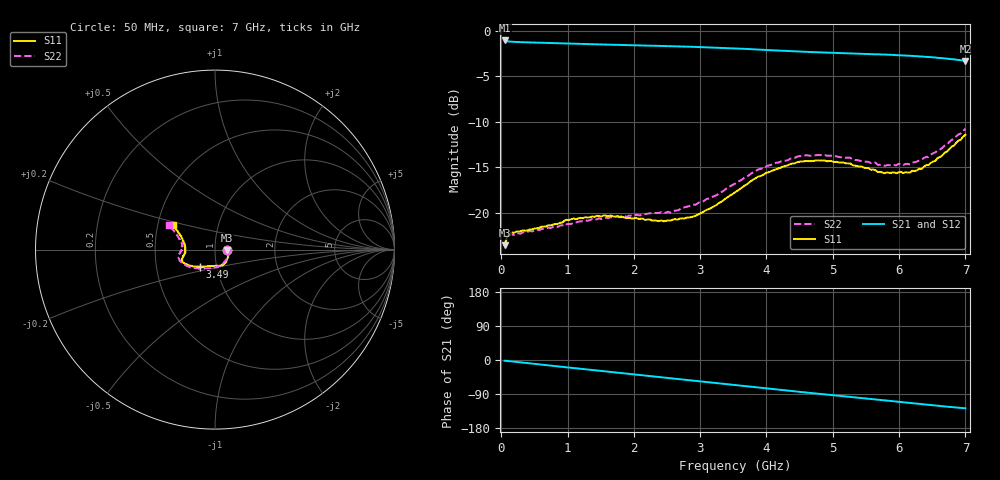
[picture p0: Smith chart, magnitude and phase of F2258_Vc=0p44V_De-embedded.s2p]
! Integrated Device Technology
! Corporate Headquarters
! 6024 Silver Creek Valley Road
! San Jose, CA 95138  USA
! Phone:  1-408-284-8200
! Toll Free:  1-800-223-1366
! Webpage:  http://www.idt.com/
! Timing and RF Division
! 515 Groton Road, Suite 102
! Westford, MA 01886-6024
! Device:  F2258
! Description: Voltage Variable RF Attenuator
! Frequency:  50.0 -  6000.00 MHz
! Package:  3x3 mm Thin QFN Plastic Package: 16 pin
! Ports:  2 RF, 2 DC
!  Pin  1  = NC
!  Pin  2  = NC
!  Pin  3  = RF2  = Port 2
!  Pin  4  = GND
!  Pin  5  = Vdd
!  Pin  6  = NC
!  Pin  7  = VCTRL
!  Pin  8  = NC
!  Pin  9  = GND
!  Pin 10  = RF1  = Port 1
!  Pin 11  = NC
!  Pin 12  = NC
!  Pin 13  = NC
!  Pin 14  = NC
!  Pin 15  = NC
!  Pin 16  = NC
! Vcntrl:  0.440 Volts
! Vdd:  +3.300 Volts
! Current:  1.096 mA
! Data:  The device was measured on a the F2258 evaluation board which has
!  individual transmission lines to the RF pins.  Data was collected
!  using a calibrated network analyzer.  The evaluation board was
!  de-embedded using a TRL calibration technique.
!  The reference plane is the edge of the package pin.
! Misc:  SN 10
!  Action Tracker AT0285
! Date Measured:  2014-12-10
! Date:  2016-01-13  MJV
! Note:
!  Integrated Device Technology supplies this data as a sample of measured
!  data at the package pin for this product.  Your particular data for this
!  product may vary.
!  Data was taken at 25 degrees C.
!  Integrated Device Technology reserves the right to change this data at anytime.
!Freq_(GHz)  S11M_(dB)  S11P_(deg)  S21M_(dB)  S21P_(deg)  S12M_(dB)  S12P_(deg)  S22M_(dB)  S22P_(deg)
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# GHz S dB R 50
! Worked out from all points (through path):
!   201 points, 50 MHz to 7 GHz, reference 50 ohm
!   highest |S21| = -1.05 dB at 50 MHz (marker M1); lowest = -3.3 dB at 7 GHz (marker M2)
!   group delay of S21, straight-line fit = 50.5 ps
!   lowest |S11| = -23.6 dB at 50 MHz (marker M3), VSWR 1.14, Z = 57.1 - j0.432 ohm
!   |S11| at or under -10 dB: start of sweep to end of sweep
!   |S22| runs from -23.7 to -10.8 dB; largest |S21 - S12| = 0.00039
!   S11 on the Smith chart (normalised r, x): 50 MHz: 1.14, -0.01; 3.49 GHz: 0.83, -0.16; 7 GHz: 0.60, +0.18
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0.05  -23.58 -3.3  -1.05 -2.0  -1.04 -2.0  -23.68 -3.1
0.08475  -22.64 -5.3  -1.13 -2.5  -1.13 -2.5  -22.77 -5.1
0.15425  -22.18 -8.2  -1.18 -3.7  -1.18 -3.7  -22.41 -8.9
0.71025  -21.38 -33.7  -1.32 -14.1  -1.32 -14.1  -21.65 -36.5
0.98825  -20.77 -46.8  -1.37 -19.4  -1.37 -19.4  -21.26 -51.9
1.2315  -20.60 -54.7  -1.43 -23.8  -1.43 -23.8  -20.94 -60.8
1.6485  -20.31 -66.0  -1.51 -31.4  -1.51 -31.4  -20.51 -73.9
2.37825  -20.92 -86.2  -1.64 -44.8  -1.64 -44.8  -20.02 -92.1
2.552  -20.88 -92.0  -1.67 -48.0  -1.67 -48.0  -20.00 -97.4
2.93425  -20.34 -108.7  -1.75 -55.1  -1.76 -55.1  -19.11 -110.9
3.49025  -17.93 -132.1  -1.91 -65.6  -1.91 -65.6  -16.94 -132.4
3.525  -17.77 -133.1  -1.92 -66.2  -1.92 -66.2  -16.80 -133.9
4.0115  -15.58 -147.8  -2.10 -75.3  -2.10 -75.2  -14.84 -149.7
4.46325  -14.44 -156.7  -2.26 -83.4  -2.26 -83.4  -13.83 -161.0
4.7065  -14.31 -160.0  -2.33 -87.7  -2.33 -87.7  -13.73 -165.3
5.2625  -14.58 -166.8  -2.48 -97.4  -2.48 -97.4  -13.95 -173.5
5.6795  -15.53 -173.3  -2.57 -104.6  -2.57 -104.6  -14.74 -179.1
5.85325  -15.61 -177.4  -2.62 -107.8  -2.63 -107.8  -14.77 176.3
6.166  -15.58 174.6  -2.73 -113.4  -2.73 -113.3  -14.69 170.2
6.33975  -15.19 168.0  -2.81 -116.5  -2.81 -116.5  -14.18 165.8
6.722  -13.27 155.6  -3.04 -123.1  -3.04 -123.1  -12.52 156.7
7  -11.42 149.7  -3.29 -127.4  -3.29 -127.4  -10.78 151.7
